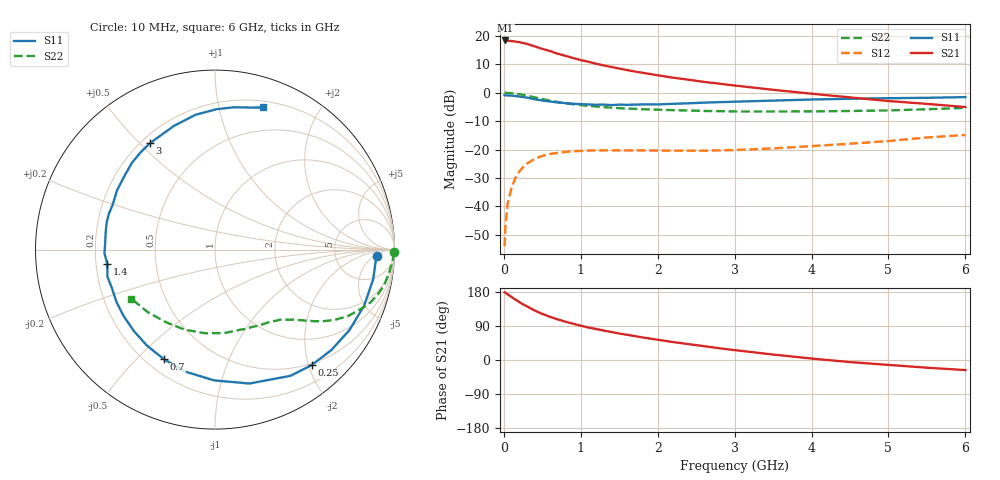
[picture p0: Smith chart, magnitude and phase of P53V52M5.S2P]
! SIEMENS Small Signal Semiconductors
! BFP183
! Si NPN RF Bipolar Junction Transistor in SOT143
! VCE = 3.5 V  IC = 2.5 mA
! Common Emitter S-Parameters:  March  1996
# GHz  S  MA  R  50
!  f  S11  S21  S12  S22
! GHz  MAG  ANG  MAG  ANG  MAG  ANG  MAG  ANG
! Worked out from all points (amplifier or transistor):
!   36 points, 10 MHz to 6 GHz, reference 50 ohm
!   highest |S21| = 18.4 dB at 20 MHz (marker M1)
!   |S21| within 3 dB of that: start of sweep to 506.5 MHz
!   unconditionally stable (mu >= 1): 1.977 GHz to 5.817 GHz
!   at 250 MHz: K = 0.14, MSG = 21.8 dB, |S12| = -26.2 dB
!   at 1.4 GHz: K = 0.74, MSG = 14.6 dB, |S12| = -20.3 dB
!   at 6 GHz: K = 0.96, MSG = 4.9 dB, |S12| = -14.9 dB
!   S11 on the Smith chart (normalised r, x): 10 MHz: 18, -7; 250 MHz: 0.47, -2.05; 700 MHz: 0.27, -0.60; 1.4 GHz: 0.25, -0.06; 3 GHz: 0.23, +0.54; 6 GHz: 0.26, +1.36
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0.01  0.9055 -2.1  8.29 178.8  0.002 85.9  0.9965 -0.8
0.02  0.8977 -4.1  8.297 177.8  0.0045 87.0  0.9967 -1.6
0.05  0.8968 -10.6  8.255 173.1  0.0114 86.7  0.9901 -4.0
0.15  0.8726 -31.1  7.923 159.5  0.0317 72.6  0.9629 -11.9
0.2  0.8562 -40.9  7.741 153.1  0.0408 67.7  0.9405 -15.4
0.25  0.8391 -50.1  7.487 146.8  0.0491 62.5  0.9145 -18.8
0.3  0.8194 -59.1  7.217 141.6  0.0565 58.0  0.8837 -21.6
0.4  0.7705 -75.6  6.549 130.7  0.0687 50.3  0.8294 -26.5
0.5  0.7286 -90.4  5.908 121.6  0.0773 43.4  0.7747 -30.3
0.6  0.6996 -103.7  5.403 113.9  0.0836 38.0  0.7262 -33.3
0.7  0.6739 -114.9  4.857 107.2  0.0874 33.7  0.6855 -35.6
0.8  0.6555 -125.4  4.459 101.1  0.0907 30.1  0.6531 -37.4
0.9  0.6408 -134.7  4.077 95.8  0.0938 27.0  0.6277 -38.9
1.1  0.6215 -152.2  3.494 85.7  0.0962 22.2  0.5863 -41.7
1.4  0.6055 -172.3  2.828 73.8  0.0971 17.8  0.5465 -45.7
1.8  0.6222 166.0  2.242 59.7  0.0966 15.7  0.5128 -51.0
2.2  0.638 148.8  1.836 47.4  0.0955 15.2  0.4935 -57.3
3  0.6949 121.5  1.338 26.1  0.0981 19.1  0.4681 -72.6
3.5  0.7261 108.4  1.125 14.4  0.1048 22.1  0.4678 -83.6
4.5  0.7822 89.4  0.827 -5.5  0.1268 24.8  0.4771 -110.7
5.5  0.814 76.5  0.636 -20.3  0.1633 23.6  0.5119 -137.1
6  0.8364 71.2  0.56 -26.6  0.1805 20.2  0.54 -149.5
